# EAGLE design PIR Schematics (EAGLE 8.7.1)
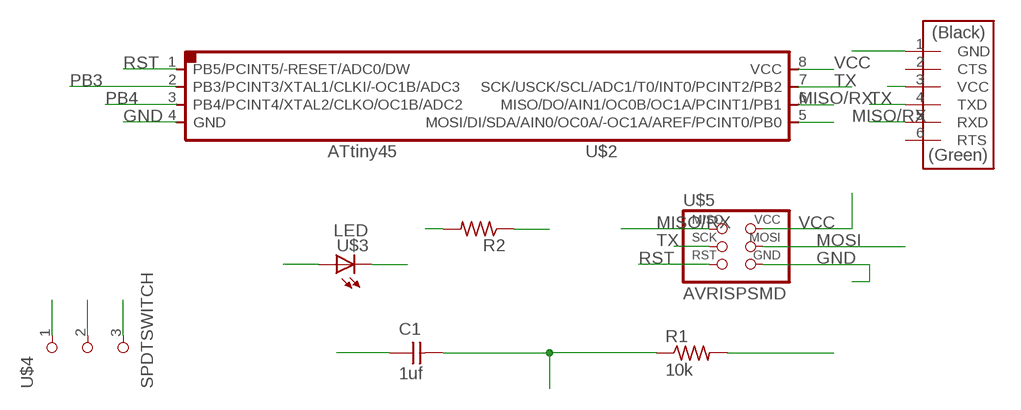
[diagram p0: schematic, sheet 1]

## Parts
C1  1uf  CAP-UNPOLARIZED  [C1206]
R1  10k  RES-US1206  [R1206]
R2  RES-US1206  [R1206]
U$1  FTDI-SMD-HEADER  [1X06SMD]
U$2  ATTINY45SI  [SOIC8]
U$3  LED  [LED1206]
U$4  SPDTSWITCH  [SPDTSWITCH]
U$5  AVRISPSMD  [2X03SMD]

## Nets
499: R2.1 U$3.1(A)
GND: C1.1 U$1.1(GND) U$2.4(GND) U$3.2(C) U$4.3 U$5.6(GND)
MISO/RX: U$1.5(RXD) U$2.6(MISO/DO/AIN1/OC0B/OC1A/PCINT1/PB1) U$5.1(MISO)
MOSI: U$2.5(MOSI/DI/SDA/AIN0/OC0A/-OC1A/AREF/PCINT0/PB0) U$5.4(MOSI)
PB3: R2.2 U$2.2(PB3/PCINT3/XTAL1/CLKI/-OC1B/ADC3)
PB4: U$2.3(PB4/PCINT4/XTAL2/CLKO/OC1B/ADC2) U$4.2
RST: R1.2 U$2.1(PB5/PCINT5/-RESET/ADC0/DW) U$5.5(RST)
TX: U$1.4(TXD) U$2.7(SCK/USCK/SCL/ADC1/T0/INT0/PCINT2/PB2) U$5.3(SCK)
VCC: C1.2 R1.1 U$1.3(VCC) U$2.8(VCC) U$4.1 U$5.2(VCC)
Unconnected: U$1.2(CTS) U$1.6(RTS)

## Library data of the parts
C1 = fab:CAP-UNPOLARIZED
R1 R2 = fab:RES-US: Resistor (US Symbol)
U$1 = fab:FTDI-SMD-HEADER
U$2 = fab:ATTINY45
U$3 = fab:LED: LED
U$4 = fab:SPDTSWITCH
U$5 = fab:AVRISP

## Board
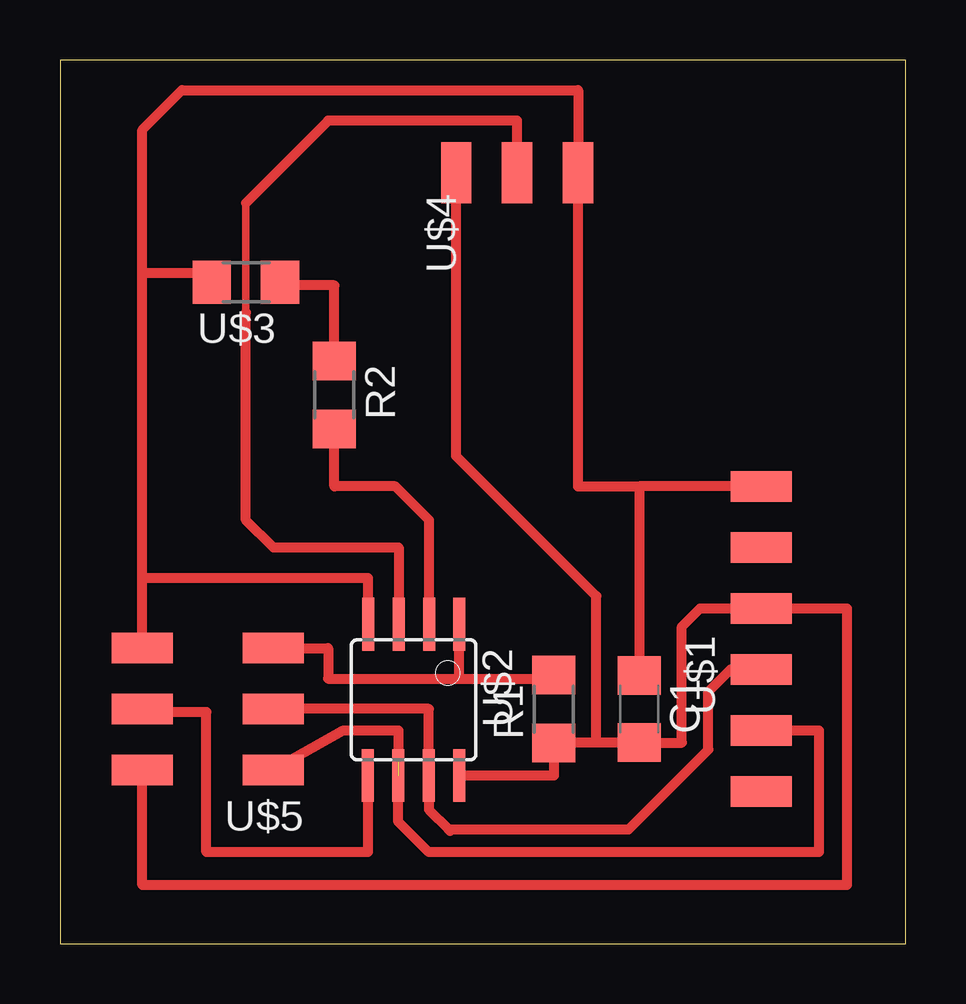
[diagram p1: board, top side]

Size 35.23 x 36.82 mm. Coordinates in mm from the lower left corner, seen from the top.
Outline: 0,0 35.23,0 35.23,36.82 0,36.82 0,0
Copper layers (1*16): Top 0.035mm / dielectric 1.5mm / Bottom 0.035mm
Design rules "fabmodule ": minimum track width 10mil, minimum drill 0.4mm, track to track 0.42mm, track to pad 0.42mm, pad to pad 0.42mm, via to via 0.42mm, smd to smd 0.42mm, copper to edge 40mil, drill to drill 0.8mm, minimum pad ring 10mil, minimum via ring 8mil, stop-mask expansion 4mil, vias tented up to drill 0mil, thermal gap 10mil

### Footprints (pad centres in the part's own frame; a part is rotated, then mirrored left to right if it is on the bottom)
C1206 = smd 1.6 x 1.8: 1 -1.4,0; 2 1.4,0
R1206 = smd 1.6 x 1.803: 1 -1.422,0; 2 1.422,0
1X06SMD = smd 2.54 x 1.27: 1 0,6.35; 2 0,3.81; 3 0,1.27; 4 0,-1.27; 5 0,-3.81; 6 0,-6.35
SOIC8 = smd 0.5 x 2.2: 1 -1.905,-3.154; 2 -0.645,-3.154; 3 0.625,-3.154; 4 1.895,-3.154; 5 1.905,3.154; 6 0.635,3.154; 7 -0.635,3.154; 8 -1.905,3.154
LED1206 = smd 1.6 x 1.803: 1 -1.422,0; 2 1.422,0
SPDTSWITCH = smd 2.54 x 1.27: 1 0.38,2.54; 2 0.38,0; 3 0.38,-2.54
2X03SMD = smd 2.54 x 1.27: 1 -2.54,2.54; 2 2.92,2.54; 3 -2.54,0; 4 2.92,0; 5 -2.54,-2.54; 6 2.92,-2.54

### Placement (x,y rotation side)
C1  24.13,9.78 270 top
R1  20.57,9.78 90 top
R2  11.43,22.86 270 top
U$1  29.21,12.7 0 top
U$2  14.73,10.16 180 top
U$3  7.75,27.56 180 top
U$4  19.05,31.75 90 top
U$5  6.35,9.78 180 top

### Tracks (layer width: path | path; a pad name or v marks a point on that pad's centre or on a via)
499
  Top 0.406: R2.1 11.43,27.43 9.3,27.43 U$3.1
GND
  Top 0.406: U$1.1 24.13,19.05 | 24.13,19.05 21.59,19.05 U$4.3 21.59,35.56 5.08,35.56 3.43,33.91 3.43,27.94 | 24.13,19.05 C1.1 | 3.43,15.24 3.43,27.94 | 3.43,15.24 12.83,15.24 12.83,13.32 U$2.4 | U$3.2 5.94,27.94 3.43,27.94 | U$5.6 3.43,15.24
MISO/RX  (1 unrouted)
  Top 0.406: U$5.1 11.81,8.89 14.1,8.89 14.1,7.62 14.1,5.08 15.37,3.81 31.62,3.81 31.62,8.89 U$1.5
MOSI
  Top 0.406: U$2.5 12.83,3.81 6.1,3.81 6.1,9.65 3.43,9.65 U$5.4
PB3
  Top 0.406: U$2.2 15.38,17.64 13.97,19.05 11.43,19.05 R2.2
PB4
  Top 0.305: 7.75,26.29 7.75,30.86
  Top 0.406: U$4.2 19.05,34.29 11.18,34.29 7.75,30.86 | U$2.3 14.11,16.51 8.89,16.51 7.75,17.65 7.75,26.29
RST
  Top 0.406: U$5.5 11.18,12.32 11.18,11.05 16.51,11.05 16.64,11.05 | 16.64,11.05 U$2.1 | 16.64,11.05 20.57,11.05 R1.2
TX
  Top 0.305: U$5.3 10.16,9.78
  Top 0.406: 16.19,4.76 15.37,5.59 U$2.7 15.37,9.78 U$5.3 | 16.19,4.76 16.26,4.7 | 16.19,4.76 23.7,4.76 27.01,8.08 27.01,10.5 27.94,11.43 U$1.4
VCC
  Top 0.305: C1.2 24.38,8.38
  Top 0.406: U$5.2 3.43,2.44 32.79,2.44 32.79,13.97 U$1.3 26.67,13.97 25.91,13.21 25.91,8.38 C1.2 | C1.2 | C1.2 22.35,8.38 | 22.35,8.38 20.57,8.38 R1.1 20.57,7.01 U$2.8 | 22.35,8.38 22.35,14.48 16.51,20.32 U$4.1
